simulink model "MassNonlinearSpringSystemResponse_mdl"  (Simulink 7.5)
settings: Solver=ode45  StartTime=0.0  StopTime=10.0  MaxStep=1e-2  RelTol=1e-3
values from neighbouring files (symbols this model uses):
  b = 0.01    [Exercises04a.m]    (also in Exercises04b.m = 0.75)
  dx0 = xe(1)    [Exercises04b.m]
  F0 = 3    [Exercises04b.m]
  k0 = 0.5    [Exercises04b.m]
  k1 = 0.25    [Exercises04b.m]
  m = 1    [Exercises04b.m]
  x0 = [70; 70]    [Exercises04a.m]    (also in Exercises04b.m = xe(2))
  xe = [c/d;a/b]    [Exercises04a.m]
libraries: cstblocks x1

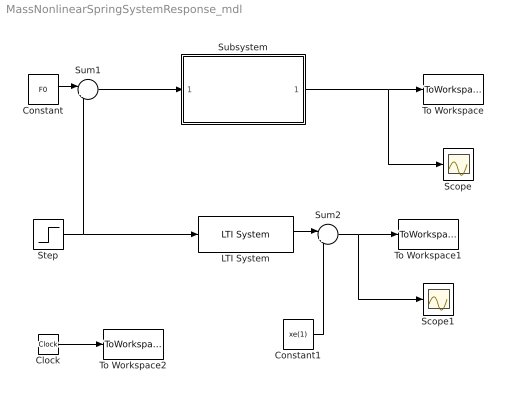
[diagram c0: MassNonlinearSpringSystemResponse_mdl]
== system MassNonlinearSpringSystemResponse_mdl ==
  Clock : Clock
  Constant : Constant  Value=F0  OutDataType=sfix(16)  OutScaling=2^0
  Constant1 : Constant  Value=xe(1)  OutDataType=sfix(16)  OutScaling=2^0
  LTI System : cstblocks/LTI System  SystemSampleTime=-1  sys=LinSys  IC=X0sl
  Scope : Scope
  Scope1 : Scope
  Step : Step  Time=2  After=0.5  SampleTime=0
  Subsystem : Subsystem
  Sum1 : Sum  Inputs=|++  OutDataType=sfix(16)  OutScaling=2^0
  Sum2 : Sum  Inputs=|++  OutDataType=sfix(16)  OutScaling=2^0
  To Workspace : ToWorkspace  VariableName=dx  SampleTime=-1  SaveFormat=Array
  To Workspace1 : ToWorkspace  VariableName=dxsl  SampleTime=-1  SaveFormat=Array
  To Workspace2 : ToWorkspace  VariableName=time  SampleTime=-1  SaveFormat=Array
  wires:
  Subsystem/1(Out1) -> To Workspace/1, Scope/1
  Step/1 -> LTI System/1, Sum1/2
  Sum1/1 -> Subsystem/1(In1)
  Constant/1 -> Sum1/1
  LTI System/1 -> Sum2/1
  Constant1/1 -> Sum2/2
  Sum2/1 -> To Workspace1/1, Scope1/1
  Clock/1 -> To Workspace2/1

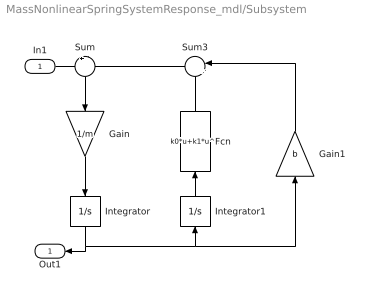
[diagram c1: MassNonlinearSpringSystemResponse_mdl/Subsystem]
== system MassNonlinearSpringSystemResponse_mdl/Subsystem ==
  In1 : Inport
  Fcn : Fcn  Expr=k0*u+k1*u^3
  Gain : Gain  Gain=1/m  ParameterDataType=sfix(16)  ParameterScaling=2^0  OutDataType=sfix(16)  OutScaling=2^0
  Gain1 : Gain  Gain=b  ParameterDataType=sfix(16)  ParameterScaling=2^0  OutDataType=sfix(16)  OutScaling=2^0
  Integrator : Integrator  InitialCondition=dx0
  Integrator1 : Integrator  InitialCondition=x0
  Sum : Sum  Inputs=+-  OutDataType=sfix(16)  OutScaling=2^0
  Sum3 : Sum  Inputs=|++  OutDataType=sfix(16)  OutScaling=2^0
  Out1 : Outport
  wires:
  Gain/1 -> Integrator/1
  Sum/1 -> Gain/1
  Integrator/1 -> Integrator1/1, Gain1/1, Out1/1
  Sum3/1 -> Sum/2
  Fcn/1 -> Sum3/2
  Gain1/1 -> Sum3/1
  Integrator1/1 -> Fcn/1
  In1/1 -> Sum/1
